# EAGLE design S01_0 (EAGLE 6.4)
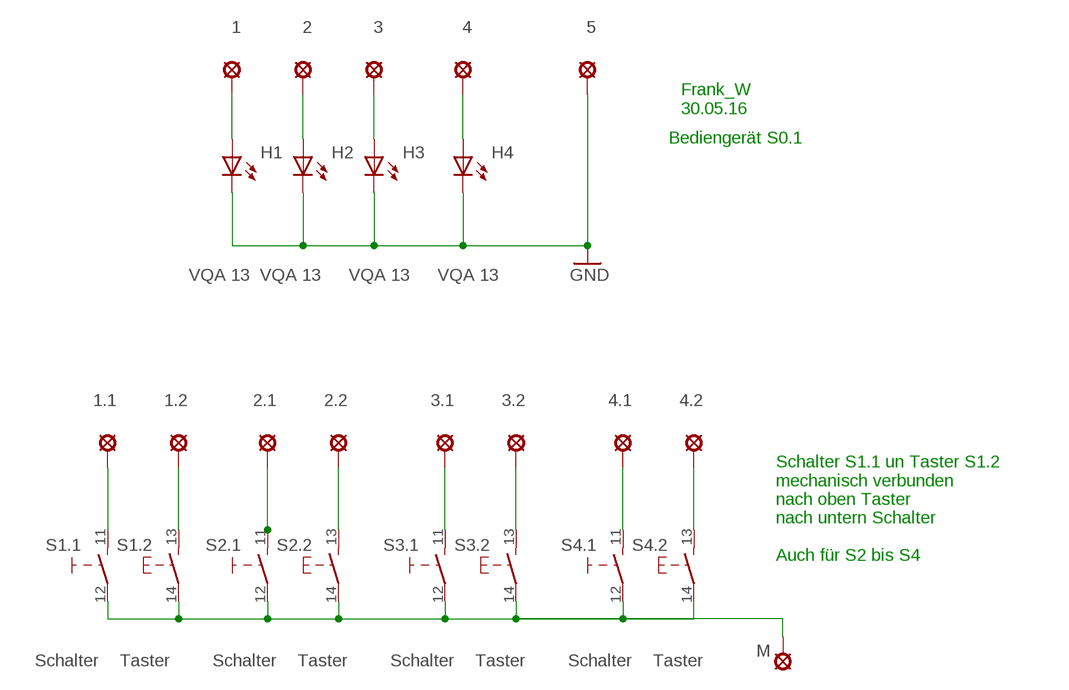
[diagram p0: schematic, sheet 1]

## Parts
1  LSP10  [LSP10]
1.1  LSP10  [LSP10]
1.2  LSP10  [LSP10]
2  LSP10  [LSP10]
2.1  LSP10  [LSP10]
2.2  LSP10  [LSP10]
3  LSP10  [LSP10]
3.1  LSP10  [LSP10]
3.2  LSP10  [LSP10]
4  LSP10  [LSP10]
4.1  LSP10  [LSP10]
4.2  LSP10  [LSP10]
5  LSP10  [LSP10]
H1  VQA 13  LED5MM  [LED5MM]
H2  VQA 13  LED5MM  [LED5MM]
H3  VQA 13  LED5MM  [LED5MM]
H4  VQA 13  LED5MM  [LED5MM]
M  LSP10  [LSP10]
S1.1  Schalter  SCHALTER_SCHLIESSER_HANDBETAETIGT  [KIPPSCHALTER_AUS]
S1.2  Taster  TASTER_SCHLIESSER  [EINTASTER]
S2.1  Schalter  SCHALTER_SCHLIESSER_HANDBETAETIGT  [KIPPSCHALTER_AUS]
S2.2  Taster  TASTER_SCHLIESSER  [EINTASTER]
S3.1  Schalter  SCHALTER_SCHLIESSER_HANDBETAETIGT  [KIPPSCHALTER_AUS]
S3.2  Taster  TASTER_SCHLIESSER  [EINTASTER]
S4.1  Schalter  SCHALTER_SCHLIESSER_HANDBETAETIGT  [KIPPSCHALTER_AUS]
S4.2  Taster  TASTER_SCHLIESSER  [EINTASTER]

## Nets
GND: 5.MP H1.K(C) H2.K(C) H3.K(C) H4.K(C)
N$1: 1.1.MP S1.1.11(CS1)
N$2: 1.2.MP S1.2.13
N$3: 2.1.MP S2.1.11(CS1)
N$4: 2.2.MP S2.2.13
N$5: 3.1.MP S3.1.11(CS1)
N$6: 3.2.MP S3.2.13
N$7: 4.1.MP S4.1.11(CS1)
N$8: 4.2.MP S4.2.13
N$9: 1.MP H1.A
N$10: 2.MP H2.A
N$11: 3.MP H3.A
N$12: 4.MP H4.A
N$14: M.MP S1.1.12(S1) S1.2.14 S2.1.12(S1) S2.2.14 S3.1.12(S1) S3.2.14 S4.1.12(S1) S4.2.14

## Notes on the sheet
- Frank_W
  30.05.16
- Bediengerät S0.1
- Schalter S1.1 un Taster S1.2
  mechanisch verbunden
  nach oben Taster
  nach untern Schalter
  
  Auch für S2 bis S4

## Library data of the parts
1 1.1 1.2 2 2.1 2.2 3 3.1 3.2 4 4.1 4.2 5 M = solpad:LSP10: SOLDER PAD
H1-H4 = led:LED: LED
S1.1 S2.1 S3.1 S4.1 = e-schalter:SCHALTER_SCHLIESSER_HANDBETAETIGT: Schließer
S1.2 S2.2 S3.2 S4.2 = e-schalter:TASTER_SCHLIESSER: Ein-Taster (Arbeitskontakt)

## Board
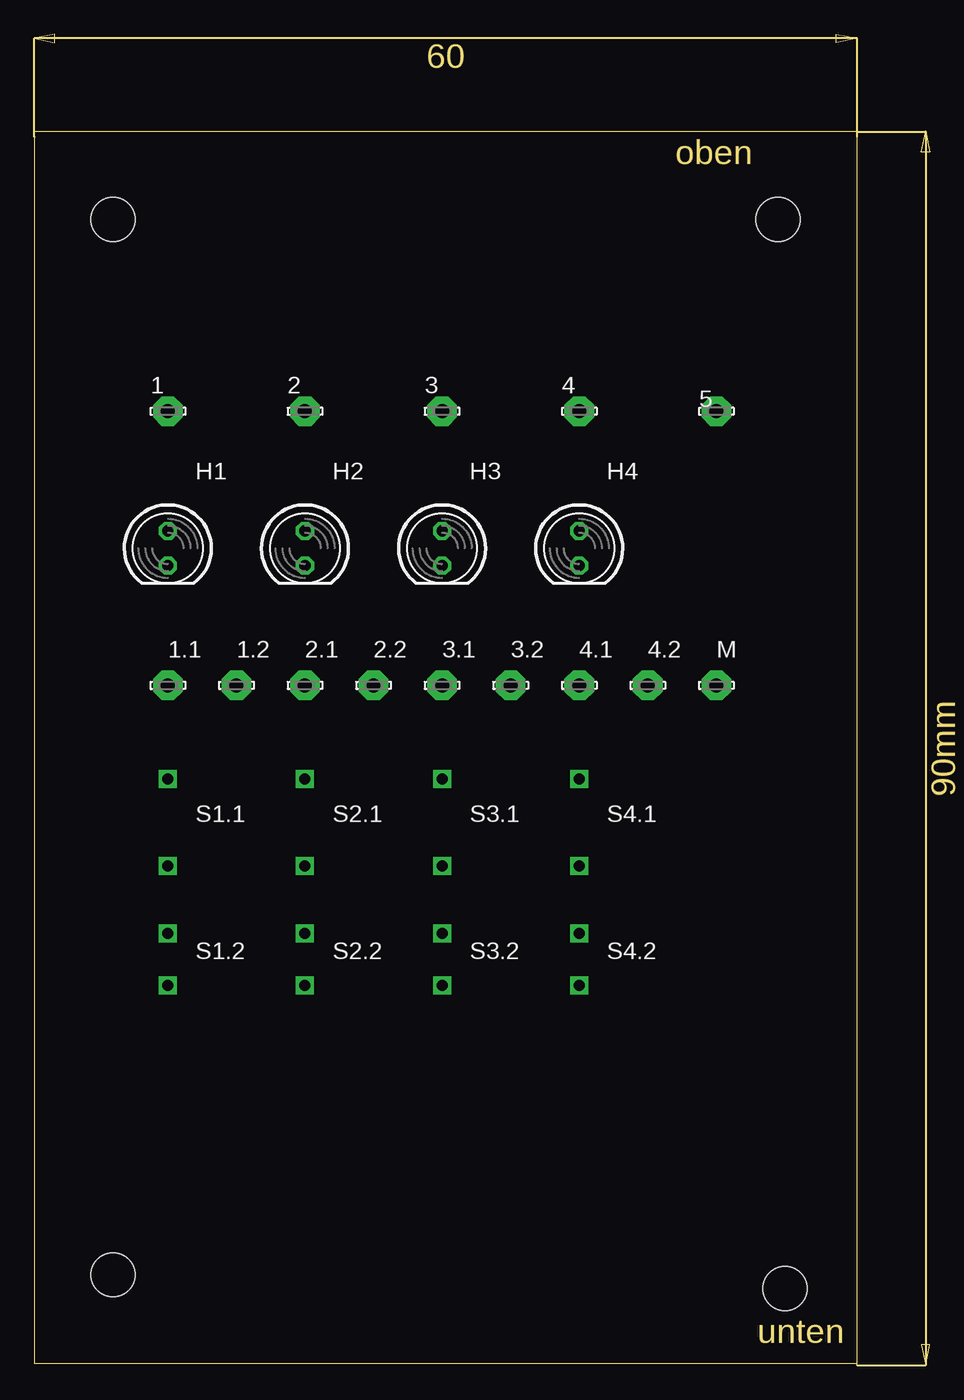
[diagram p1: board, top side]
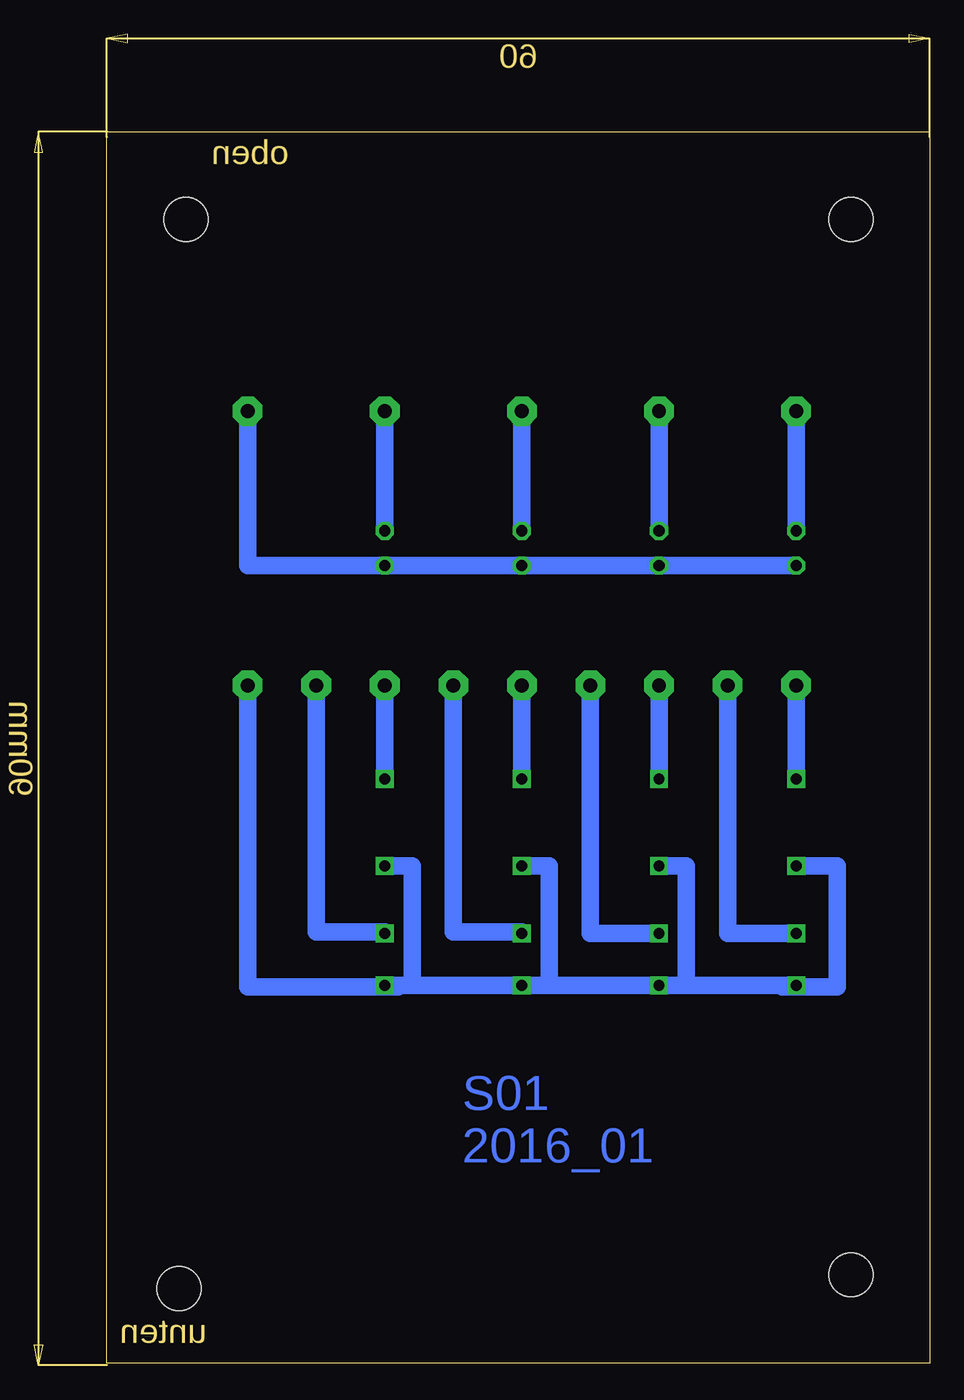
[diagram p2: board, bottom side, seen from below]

Size 65.3 x 97.1 mm. Coordinates in mm from the lower left corner, seen from the top.
Outline: 0,90 0,0.16 60,0.16 60,90 0,90
Copper layers (1*16): Top 0.035mm / dielectric 1.5mm / Bottom 0.035mm
Design rules "default *": minimum track width 20mil, minimum drill 24mil, track to track 8mil, track to pad 8mil, pad to pad 8mil, via to via 8mil, smd to smd 8mil, copper to edge 40mil, drill to drill 8mil, minimum pad ring 10mil, minimum via ring 8mil, stop-mask expansion 4mil, vias tented up to drill 0mil, thermal gap 20mil
Holes 3.2 mm at 54.74,5.6 5.74,6.6 5.74,83.6 54.24,83.6

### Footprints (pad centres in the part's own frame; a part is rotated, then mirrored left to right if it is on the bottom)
LSP10 = drill 1.016 pad 2.159 octagon: MP 0,0
LED5MM = drill 0.813 octagon: A -1.27,0; K 1.27,0
KIPPSCHALTER_AUS = drill 0.8 square: 11 0,3.175; 12 0,-3.175
EINTASTER = drill 0.8 square: 13 0,1.905; 14 0,-1.905

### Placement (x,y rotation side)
1  9.74,69.6 0 top
1.1  9.74,49.6 0 top
1.2  14.74,49.6 0 top
2  19.74,69.6 0 top
2.1  19.74,49.6 0 top
2.2  24.74,49.6 0 top
3  29.74,69.6 0 top
3.1  29.74,49.6 0 top
3.2  34.74,49.6 0 top
4  39.74,69.6 0 top
4.1  39.74,49.6 0 top
4.2  44.74,49.6 0 top
5  49.74,69.6 0 top
H1  9.74,59.6 270 top
H2  19.74,59.6 270 top
H3  29.74,59.6 270 top
H4  39.74,59.6 270 top
M  49.74,49.6 0 top
S1.1  9.74,39.6 0 top
S1.2  9.74,29.6 0 top
S2.1  19.74,39.6 0 top
S2.2  19.74,29.6 0 top
S3.1  29.74,39.6 0 top
S3.2  29.74,29.6 0 top
S4.1  39.74,39.6 0 top
S4.2  39.74,29.6 0 top

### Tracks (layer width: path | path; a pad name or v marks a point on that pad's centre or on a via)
GND
  Bottom 1.27: H1.K H2.K H3.K H4.K 49.74,58.33 5.MP
N$1
  Bottom 1.27: S1.1.11 1.1.MP
N$2
  Bottom 1.27: S1.2.13 14.74,31.51 1.2.MP
N$3
  Bottom 1.27: S2.1.11 2.1.MP
N$4
  Bottom 1.27: S2.2.13 24.74,31.51 2.2.MP
N$5
  Bottom 1.27: S3.1.11 3.1.MP
N$6
  Bottom 1.27: 3.2.MP 34.74,31.6 29.74,31.6 S3.2.13
N$7
  Bottom 1.27: S4.1.11 4.1.MP
N$8
  Bottom 1.27: 4.2.MP 44.74,31.6 39.74,31.6 S4.2.13
N$9
  Bottom 1.27: H1.A 1.MP
N$10
  Bottom 1.27: H2.A 2.MP
N$11
  Bottom 1.27: H3.A 3.MP
N$12
  Bottom 1.27: H4.A 4.MP
N$14
  Bottom 1.27: S1.2.14 10.74,27.7 | 10.74,27.7 17.74,27.7 | 17.74,27.7 S2.2.14 27.74,27.7 | 27.74,27.7 S3.2.14 37.74,27.7 | 37.74,27.7 38.74,27.7 | 38.74,27.7 S4.2.14 | S1.1.12 6.74,36.43 6.74,27.6 10.74,27.6 10.74,27.7 | S2.1.12 17.74,36.43 17.74,27.7 | S3.1.12 27.74,36.43 27.74,27.7 | S4.1.12 37.74,36.43 37.74,27.7 | M.MP 49.74,27.6 38.74,27.6 38.74,27.7

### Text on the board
Bottom: S01 / 2016_01
Dimension: oben | unten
